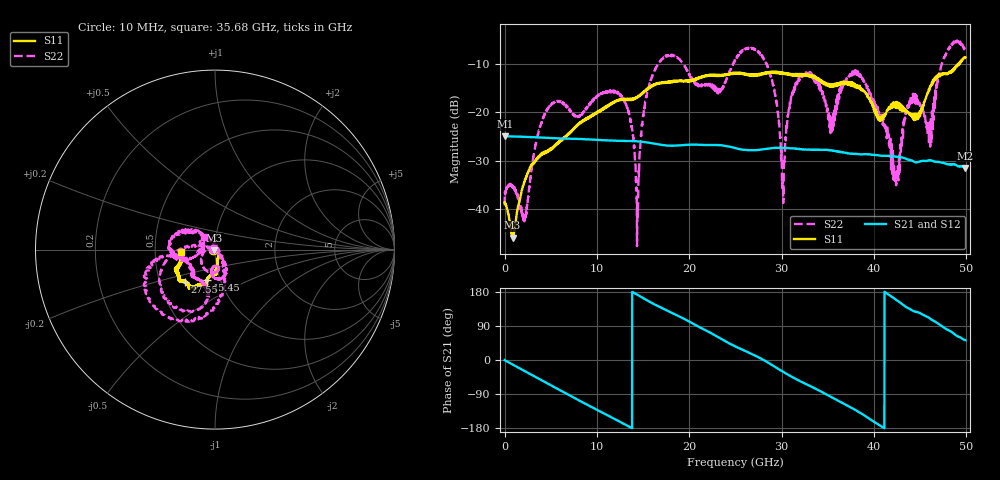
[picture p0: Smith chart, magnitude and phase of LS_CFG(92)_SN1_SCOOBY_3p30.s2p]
!Keysight Technologies,N5245B,MY58422026,A.13.80.08
!Date: Thursday, March 19, 2020 23:55:57
!Correction: S11(Full 2 Port(1,2))
!S21(Full 2 Port(1,2))
!S12(Full 2 Port(1,2))
!S22(Full 2 Port(1,2))
!S2P File: Measurements: S11, S21, S12, S22:
# Hz S DB R 50.0
!freq dBS11 angS11 dBS21 angS21 dBS12 angS12 dBS22 angS22
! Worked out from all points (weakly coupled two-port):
!   4991 points, 10 MHz to 49.91 GHz, reference 50 ohm
!   highest |S21| = -24.90 dB at 20 MHz (marker M1); lowest = -31.5 dB at 49.91 GHz (marker M2)
!   lowest |S11| = -46.0 dB at 870 MHz (marker M3), VSWR 1.01, Z = 49.7 - j0.367 ohm
!   |S11| at or under -10 dB: start of sweep to 49.12 GHz; 49.17112 GHz to 49.22245 GHz (51.33 MHz wide, 0.104 % of centre)
!   |S22| runs from -47.7 to -5.1 dB; largest |S21 - S12| = 0.00058
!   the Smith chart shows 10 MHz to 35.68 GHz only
!   S11 on the Smith chart (normalised r, x): 10 MHz: 0.98, -0.01; 15.45 GHz: 0.87, -0.30; 27.55 GHz: 0.67, -0.26; 35.68 GHz: 0.68, -0.02
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1e7  -38.68 -166.3  -24.90 -0.3  -24.89 -0.3  -39.24 175.7
2e7  -38.57 -176.0  -24.90 -0.4  -24.90 -0.4  -37.18 -178.1
8.7e8  -45.97 -132.7  -24.97 -11.8  -24.97 -11.8  -35.34 -112.0
2.15e9  -34.53 -53.1  -25.05 -28.9  -25.04 -28.9  -42.55 31.8
4.51e9  -28.11 -59.7  -25.24 -60.1  -25.24 -60.1  -19.87 -137.7
8.33e9  -22.10 -80.3  -25.51 -110.1  -25.51 -110.0  -20.41 -94.3
1.267e10  -17.40 -87.9  -25.89 -165.0  -25.88 -164.9  -16.59 -67.3
1.436e10  -16.91 -99.3  -25.97 172.5  -25.96 172.7  -45.38 -82.6
1.545e10  -15.25 -105.3  -26.22 157.3  -26.21 157.4  -15.76 174.3
1.665e10  -14.02 -103.9  -26.60 141.5  -26.60 141.6  -9.92 -158.6
2.496e10  -11.92 -124.5  -27.34 36.1  -27.33 36.3  -9.27 -167.7
2.755e10  -12.09 -132.9  -27.75 6.5  -27.75 6.8  -7.61 -109.2
3.014e10  -11.92 -143.0  -27.37 -30.5  -27.38 -30.2  -34.21 26.5
3.116e10  -12.11 -146.2  -27.45 -44.9  -27.46 -44.5  -15.87 142.5
3.328e10  -12.46 -155.7  -27.71 -71.2  -27.71 -70.7  -12.16 -173.9
3.568e10  -14.36 -176.6  -27.96 -101.6  -27.90 -101.1  -20.03 132.5
3.816e10  -14.88 176.3  -28.62 -134.3  -28.57 -134.3  -11.38 -175.1
4.16e10  -19.03 108.7  -29.01 172.6  -29.03 172.6  -25.04 71.3
4.245e10  -18.04 107.3  -29.18 158.3  -29.19 158.3  -34.52 -177.6
4.39e10  -20.27 80.4  -29.84 134.4  -29.87 134.5  -17.51 -31.7
4.601e10  -15.37 8.7  -29.88 110.6  -29.89 110.8  -23.10 114.0
4.991e10  -8.57 -13.0  -31.48 52.2  -31.51 52.3  -7.31 -14.8
